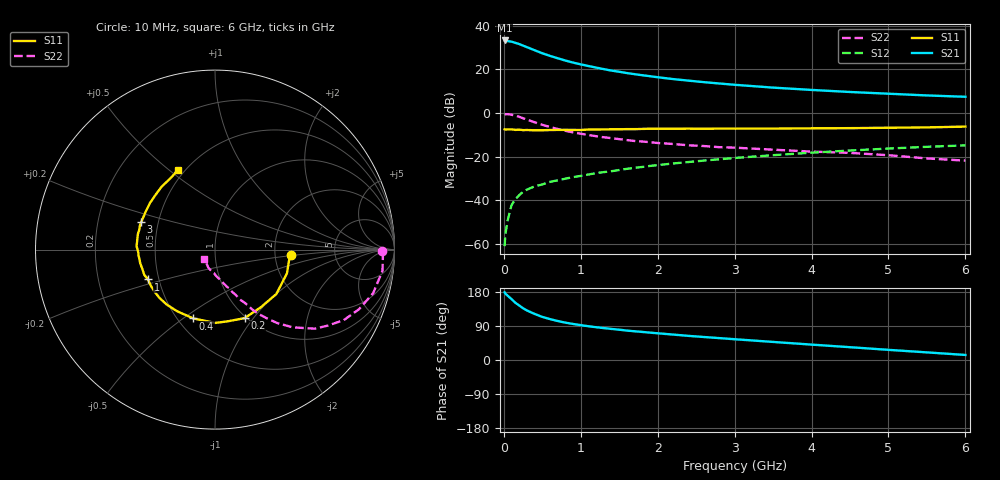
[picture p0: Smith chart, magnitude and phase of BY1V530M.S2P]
! SIEMENS Small Signal Semiconductors
! BFY420
! Si NPN RF SIEGET Grounded Emitter Transistor in MICRO-X
! VCE = 1.5 V  IC = 30 mA
! Common Emitter S-Parameters:  October  1996
# GHz  S  MA  R  50
!  f  S11  S21  S12  S22
! GHz  MAG  ANG  MAG  ANG  MAG  ANG  MAG  ANG
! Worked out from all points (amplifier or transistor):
!   36 points, 10 MHz to 6 GHz, reference 50 ohm
!   highest |S21| = 33.2 dB at 10 MHz (marker M1)
!   |S21| within 3 dB of that: start of sweep to 295.6 MHz
!   unconditionally stable (mu >= 1): start of sweep to 11.67 MHz; 1.5 GHz to end of sweep
!   at 250 MHz: K = 0.38, MSG = 33.4 dB, |S12| = -36.0 dB
!   at 1.4 GHz: K = 0.99, MSG = 23.0 dB, |S12| = -26.6 dB
!   at 6 GHz: K = 1.08, MAG = 9.4 dB, |S12| = -14.8 dB
!   S11 on the Smith chart (normalised r, x): 10 MHz: 2.45, -0.19; 200 MHz: 0.98, -0.91; 400 MHz: 0.60, -0.55; 1 GHz: 0.44, -0.17; 3 GHz: 0.40, +0.15; 6 GHz: 0.46, +0.53
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0.01  0.4232 -4.2  45.61 178.6  0.0009 113.8  0.9329 -0.6
0.02  0.417 -8.1  45.36 175.3  0.0017 95.5  0.9362 -2.2
0.05  0.4222 -18.4  44.12 169.6  0.0035 83.3  0.9406 -7.2
0.1  0.4218 -36.0  42.79 160.6  0.0078 78.0  0.914 -15.4
0.15  0.4104 -51.7  40.22 151.0  0.0107 73.6  0.8684 -22.5
0.2  0.4158 -66.6  37.73 143.8  0.0132 70.1  0.818 -28.7
0.25  0.4059 -79.6  34.76 136.5  0.0158 64.4  0.7586 -33.9
0.3  0.4085 -89.9  32.06 130.7  0.0177 64.8  0.7092 -38.4
0.4  0.4021 -107.5  27.26 121.6  0.021 61.0  0.6126 -45.0
0.5  0.4029 -121.4  23.23 113.7  0.0232 60.2  0.5368 -49.7
0.6  0.4079 -131.4  20.25 107.9  0.0266 59.5  0.4774 -53.1
0.8  0.4106 -145.5  15.83 98.6  0.0315 58.7  0.3912 -58.2
1  0.4089 -156.0  12.94 92.0  0.0364 60.0  0.3359 -61.1
1.1  0.4187 -160.5  11.87 89.1  0.0392 60.3  0.3142 -63.1
1.4  0.4238 -170.4  9.322 82.0  0.0467 60.6  0.2657 -66.6
1.6  0.4277 -175.7  8.188 77.6  0.0529 59.4  0.24 -69.2
2.2  0.4367 172.2  5.97 67.1  0.07 57.5  0.1957 -75.6
3  0.4388 159.5  4.419 54.8  0.0936 52.6  0.1612 -83.0
3.5  0.4401 151.5  3.804 47.7  0.1084 48.8  0.1449 -88.2
4.5  0.4504 137.1  3.023 33.8  0.1387 39.9  0.1224 -98.5
5.5  0.4684 122.0  2.52 20.1  0.1686 30.1  0.0914 -120.6
6  0.4885 115.2  2.349 13.3  0.182 24.9  0.0814 -138.4
